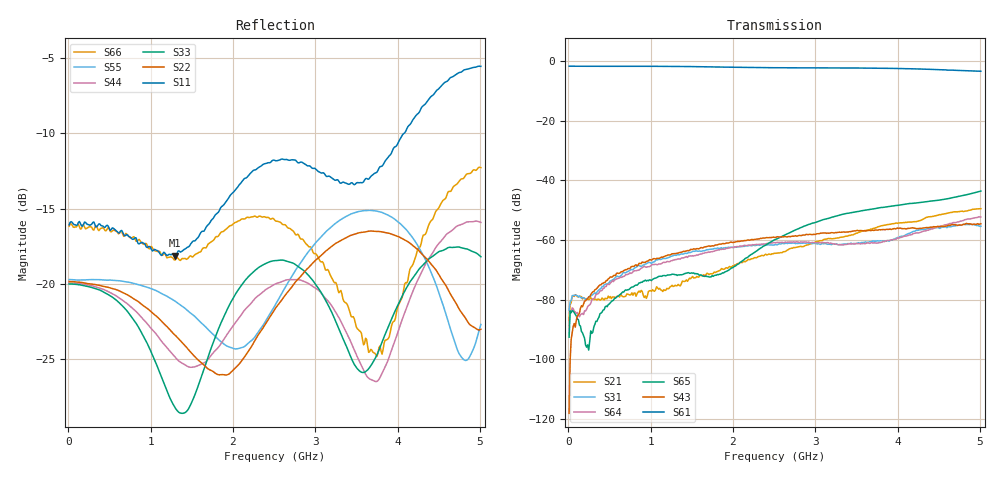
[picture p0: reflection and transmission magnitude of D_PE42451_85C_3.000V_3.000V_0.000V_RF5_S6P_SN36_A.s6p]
! Device ID: PE42451
! Serial: 36
! Insertion: A
! Temp: 85C
! VDD: 3.000
! Control_Hi: 100.000
! Control_Lo: 0.000
! Logic State: RF5
! Port 1: RFC
! Port 2: RF1
! Port 3: RF2
! Port 4: RF3
! Port 5: RF4
! Port 6: RF5
! V1 = 3.00
! V2 = 0.00
! V3 = 3.00
! V4 = 0.00
! IDD: 1.439110e-05
#  Hz  S  RI  R  50
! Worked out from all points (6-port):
!   401 points, 10 MHz to 5.01 GHz, reference 50 ohm
!   strongest paths, dB at 10 MHz, 1.26 GHz, 2.51 GHz, 3.76 GHz, 5.01 GHz:
!     S61: -1.7, -1.7, -2.2, -2.3, -3.4
!     S43: -118.1, -64.6, -59.1, -56.6, -54.5
!     S65: -92.6, -71.4, -59.9, -49.3, -43.5
!     S64: -88.6, -66.9, -60.8, -61.0, -52.2
!     S31: -83.5, -65.4, -61.5, -60.3, -55.4
!     S21: -87.0, -75.1, -64.4, -55.5, -49.5
!   lowest |S11| = -18.1 dB at 1.298 GHz (marker M1), VSWR 1.28, Z = 55.1 - j12.1 ohm
!   |S11| at or under -10 dB: start of sweep to 4.078 GHz
